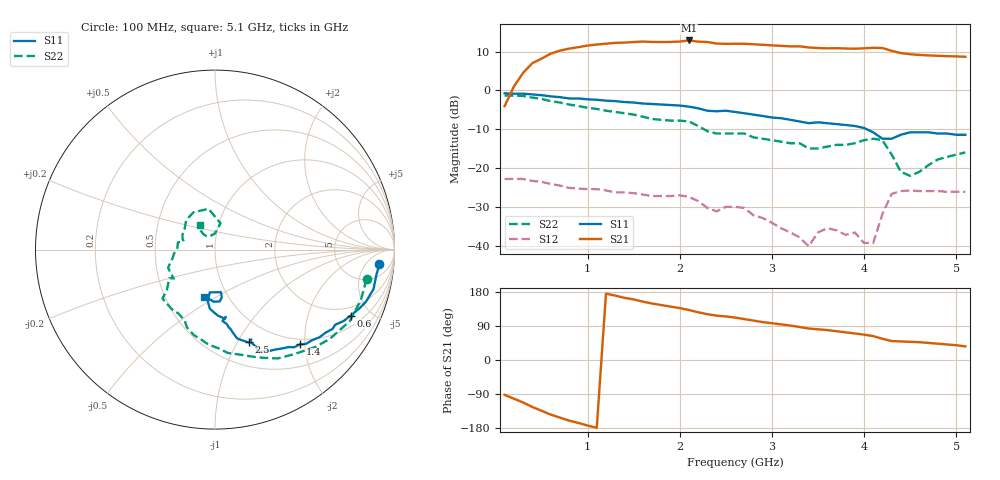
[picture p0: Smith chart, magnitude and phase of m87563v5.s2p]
!  MGA-87563 S PARAMETERS
!  Vd = 5 V  LAST UPDATED 12-21-94
# ghz s ma r 50
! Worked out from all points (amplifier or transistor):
!   51 points, 100 MHz to 5.1 GHz, reference 50 ohm
!   highest |S21| = 12.8 dB at 2.1 GHz (marker M1)
!   |S21| within 3 dB of that: 650.4 MHz to 4.357 GHz (3.707 GHz wide, 148 % of centre)
!   unconditionally stable (mu >= 1): 1.473 GHz to end of sweep
!   at 900 MHz: K = 0.64, MSG = 18.2 dB, |S12| = -25.2 dB
!   at 2.6 GHz: K = 2.62, MAG = 13.9 dB, |S12| = -29.9 dB
!   at 5.1 GHz: K = 3.36, MAG = 9.2 dB, |S12| = -26.0 dB
!   lowest NFmin = 1.52 dB at 1.4 GHz
!   S11 on the Smith chart (normalised r, x): 100 MHz: 11, -12; 600 MHz: 1.50, -3.76; 1.4 GHz: 0.90, -1.91; 2.5 GHz: 0.75, -1.12; 5.1 GHz: 0.78, -0.44
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0.1  0.92 -5.0  0.63 -92.0  0.073 -7.0  0.86 -11.0
0.3  0.91 -14.0  1.68 -112.0  0.073 -13.0  0.85 -28.0
0.4  0.89 -19.0  2.24 -124.0  0.069 -19.0  0.81 -38.0
0.6  0.84 -26.0  2.97 -144.0  0.063 -24.0  0.73 -53.0
0.8  0.79 -32.0  3.45 -160.0  0.056 -27.0  0.66 -66.0
1  0.77 -37.0  3.77 -173.0  0.054 -28.0  0.6 -77.0
1.2  0.74 -43.0  3.99 175.0  0.052 -32.0  0.55 -88.0
1.4  0.71 -48.0  4.12 164.0  0.049 -34.0  0.51 -98.0
1.6  0.68 -53.0  4.25 154.0  0.046 -37.0  0.46 -110.0
1.8  0.66 -57.0  4.19 145.0  0.044 -37.0  0.42 -116.0
2.1  0.62 -67.0  4.39 132.0  0.043 -52.0  0.4 -137.0
2.4  0.54 -68.0  4.01 117.0  0.028 -44.0  0.28 -145.0
2.5  0.55 -70.0  3.97 115.0  0.032 -42.0  0.28 -146.0
2.6  0.53 -73.0  3.98 112.0  0.032 -49.0  0.28 -152.0
2.9  0.47 -78.0  3.86 100.0  0.023 -57.0  0.24 -169.0
3.4  0.38 -81.0  3.57 83.0  0.01 -5.0  0.18 165.0
3.5  0.39 -82.0  3.51 81.0  0.015 -2.0  0.18 165.0
4.1  0.29 -98.0  3.53 63.0  0.011 54.0  0.24 120.0
4.2  0.24 -97.0  3.51 56.0  0.026 75.0  0.23 99.0
4.3  0.24 -82.0  3.23 50.0  0.047 51.0  0.15 78.0
4.5  0.29 -85.0  2.92 48.0  0.052 22.0  0.08 111.0
5.1  0.27 -103.0  2.71 36.0  0.05 -3.0  0.16 122.0
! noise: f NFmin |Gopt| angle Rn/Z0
0.1  3.57  0.72  -8  2.72
0.6  2.45  0.7  8  1.67
1.2  1.56  0.68  20  0.78
1.7  1.55  0.66  31  0.68
2.3  1.59  0.64  40  0.62
2.8  1.64  0.61  46  0.58
3.4  1.8  0.55  53  0.57
3.9  1.93  0.5  60  0.57
4.5  2.02  0.45  70  0.54
5.1  2.04  0.43  81  0.46
